FUNCTION_BLOCK FB_DO_IED_LD1_ATCC1_TapChg EXTENDS FB_AcsiCommonControllableDataClass
VAR_INPUT
	valWTr: FB_AcsiDATypeValWithTrans := (fc:=ACSI_FC_ST, TrgOp:=ACSI_TrgOp_dchg, bLinkResult:=THIS^.AddDataToContainer(ipData:=valWTr));
	q: FB_AcsiDATypeQuality := (fc:=ACSI_FC_ST, TrgOp:=ACSI_TrgOp_qchg, bLinkResult:=THIS^.AddDataToContainer(ipData:=q));
	t: FB_AcsiDATypeTimeStamp := (fc:=ACSI_FC_ST, bLinkResult:=THIS^.AddDataToContainer(ipData:=t));
	stSeld: FB_AcsiBATypeBOOLEAN := (fc:=ACSI_FC_ST, TrgOp:=ACSI_TrgOp_dchg, bLinkResult:=THIS^.AddDataToContainer(ipData:=stSeld));
	persistent_: FB_AcsiBATypeBOOLEAN := (sObjectName:='persistent', fc:=ACSI_FC_CF, TrgOp:=ACSI_TrgOp_dchg, bLinkResult:=THIS^.AddDataToContainer(ipData:=persistent_));
	ctlModel: FB_AcsiDATypeCtlModels := (fc:=ACSI_FC_CF, TrgOp:=ACSI_TrgOp_dchg, eValue:=E_AcsiCtlModels.DirectWithEnhancedSecurity, bLinkResult:=THIS^.AddDataToContainer(ipData:=ctlModel));
	Oper: FB_AcsiCDC_Oper_CODEDENUM := (fc:=ACSI_FC_CO, bLinkResult:=THIS^.AddDataToContainer(ipData:=Oper));
	
	fbControl: FB_DirectControl := (ipCtrl:=THIS^.AddServerJob(ipEvent:=fbControl, ipCompletion:=fbControl), eType:=E_AcsiCDCType.BSC, ipBehVal:=fbIED.IEDLD1.ATCC1.Beh.stVal);
END_VAR
VAR
END_VAR

END_FUNCTION_BLOCK
